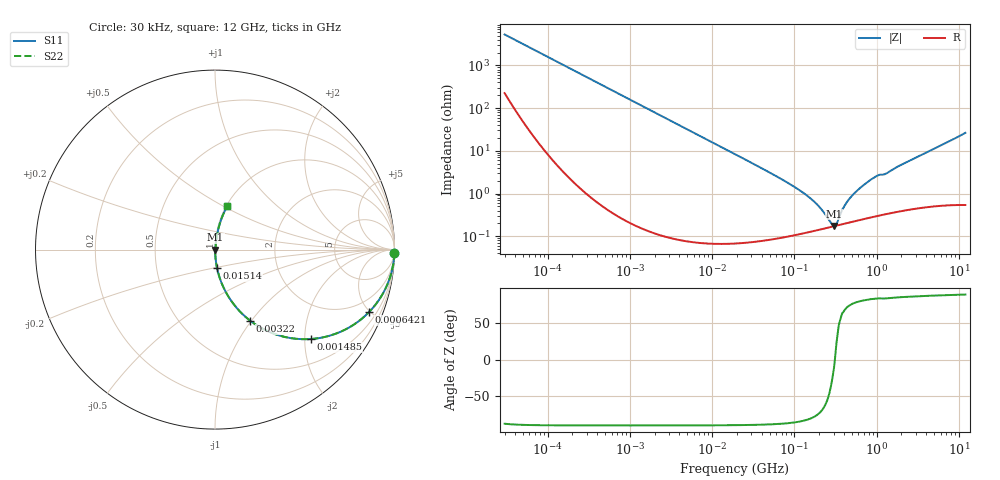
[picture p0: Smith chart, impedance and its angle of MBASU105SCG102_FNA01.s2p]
! MBASU105SCG102_FNA01  S-PARAMETER MODEL  ( General Type )
! Model Generated by TAIYO YUDEN Corporation (http://www.ty-top.com)
! Version 1.0
! TAIYO YUDEN Control No. 130207
! Copyright(c) 2013 TAIYO YUDEN CO.,LTD. All Rights Reserved.
! Product Description (link to TY-COMPAS)
! https://ds.yuden.co.jp/TYCOMPAS/or/detail?pn=MBASU105SCG102JFNA01&u=M
! Products Name : Multilayer Ceramic Capacitors
! Characteristics :
!  Capacitance : 1000 pF , Rated Voltage : 50V , TCC : CG / C0G
!  Case Size : 1.0 x 0.5 / 0.039 x 0.02 [mm/inch] , Thickness : 0.5 / 0.02 [mm/inch]
!  (Conditions: Temperature = 25 degC , DC Bias Current/Voltage = 0A / 0V)
! External Node Assignments :
!  1  o---| |---o  2
! GND o---------o GND
! Frequency Range : 30000Hz  -  12GHz  [ 401 STEP ]
# MHz S RI R 50
! Freq[MHz].  S11 Real  S11 Imag  S21 Real  S21 Imag  S12 Real  S12 Imag  S22 Real  S22 Imag
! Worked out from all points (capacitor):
!   401 points, 30 kHz to 12 GHz, reference 50 ohm
!   read as one part in series: C = 1 nF near 32 kHz
!   lowest |Z| = 174 mohm at 303.8 MHz (marker M1)
!   series resonance near 310.8 MHz, so ESL is about 260 pH
!   S11 on the Smith chart (normalised r, x): 30 kHz: open; 642.1 kHz: 1.01, -4.96; 1.485 MHz: 1.00, -2.14; 3.22 MHz: 1.00, -0.99; 15.14 MHz: 1.00, -0.21; 12 GHz: 1.01, +0.53
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0.03  0.9989 -0.0188  0.00115 0.0188  0.00115 0.0188  0.9989 -0.0188
0.105517  0.9953 -0.066  0.0047 0.066  0.0047 0.066  0.9953 -0.066
0.260295  0.9736 -0.1592  0.0264 0.1592  0.0264 0.1592  0.9736 -0.1592
0.642112  0.8596 -0.3467  0.1404 0.3467  0.1404 0.3467  0.8596 -0.3467
1.485061  0.5344 -0.4981  0.4656 0.4981  0.4656 0.4981  0.5344 -0.4981
2.258455  0.3319 -0.4701  0.6681 0.4701  0.6681 0.4701  0.3319 -0.4701
3.22009  0.1966 -0.3966  0.8034 0.3966  0.8034 0.3966  0.1966 -0.3966
6.13721  0.0635 -0.2425  0.9365 0.2425  0.9365 0.2425  0.0635 -0.2425
15.13963  0.0115 -0.1036  0.9885 0.1036  0.9885 0.1036  0.0115 -0.1036
18.97367  0.00759 -0.0829  0.9924 0.0829  0.9924 0.0829  0.00759 -0.0829
80.98098  0.0013 -0.0183  0.9987 0.0183  0.9987 0.0183  0.0013 -0.0183
164.6252  0.00134 -0.00698  0.9987 0.00698  0.9987 0.00698  0.00134 -0.00698
213.0775  0.00147 -0.00401  0.9985 0.00401  0.9985 0.00401  0.00147 -0.00401
284.8288  0.00166 -0.000972  0.9983 0.000972  0.9983 0.000972  0.00166 -0.000972
303.8045  0.00171 -0.000318  0.9983 0.000318  0.9983 0.000318  0.00171 -0.000318
334.6645  0.00179 0.0012  0.9982 -0.0012  0.9982 -0.0012  0.00179 0.0012
406.107  0.00198 0.0047  0.998 -0.0047  0.998 -0.0047  0.00198 0.0047
542.8588  0.00234 0.0101  0.9977 -0.0101  0.9977 -0.0101  0.00234 0.0101
939.2353  0.00342 0.0235  0.9966 -0.0235  0.9966 -0.0235  0.00342 0.0235
1428.372  0.00444 0.0321  0.9956 -0.0321  0.9956 -0.0321  0.00444 0.0321
5023.914  0.0172 0.1098  0.9828 -0.1098  0.9828 -0.1098  0.0172 0.1098
12000  0.0696 0.2445  0.9304 -0.2445  0.9304 -0.2445  0.0696 0.2445
